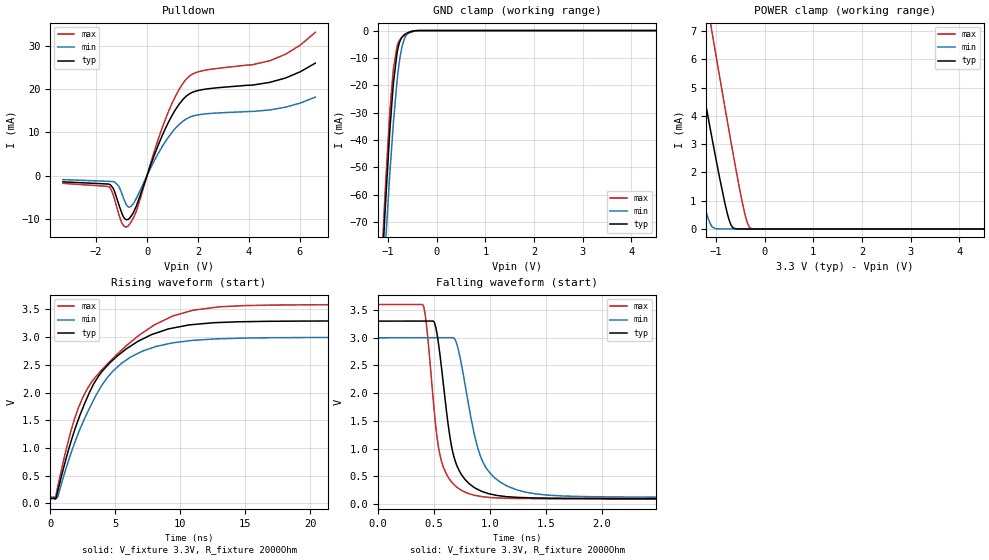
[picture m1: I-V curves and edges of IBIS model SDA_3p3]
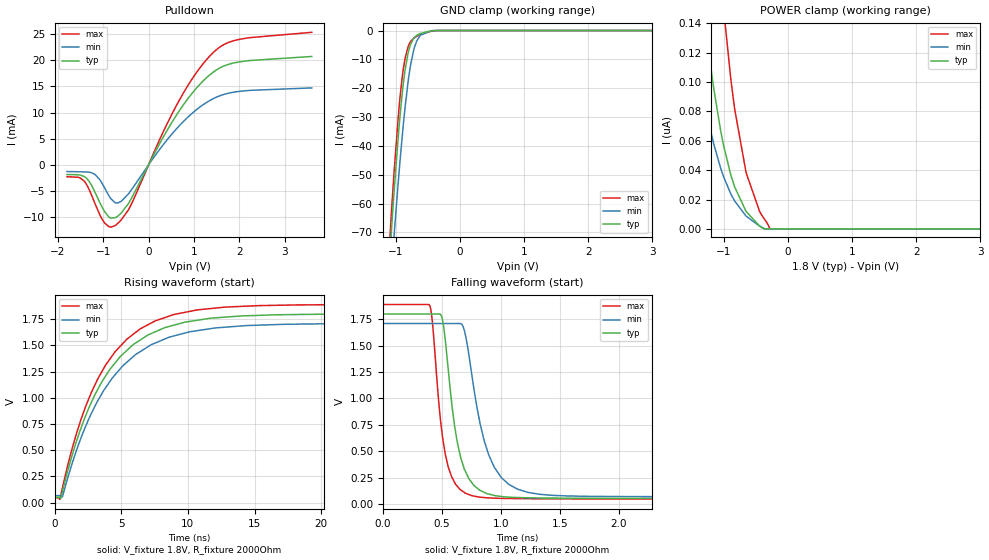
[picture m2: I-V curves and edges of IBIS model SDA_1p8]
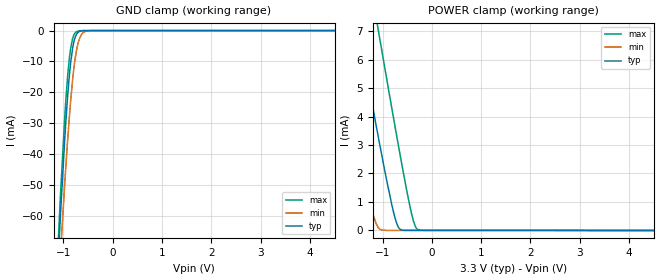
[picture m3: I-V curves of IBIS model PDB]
|Texas Instruments Incorporated
| Marketing part#   Digital Voltage Range   Package-type   #pins
| DS90UB940N-Q1   1.71V-3.6V   QFN   64
[IBIS Ver]   4.1
[File name]   ds90ub940n_q1.ibs
[File Rev]   1.0
[Date]   03/19/2019
[Source]
| Texas Instruments Incorporated.
| 12500 TI Blvd
| Dallas, TX -75243
[Notes]   Revision History:
| Rev 1.0: 03/19/2019
| - Initial version of the model
| - Model generated from simulations in TISPICE
| - C_comp although listed in numerical order of value are
|   obtained from varying PVT conditions. For PVT conditions for
|   each specific value refer the buffer description under
|   respective [Model]. IBIS model user is responsible for using
|   appropriate C_comp to simulate for Signal Integrity.
| - Warnings regarding combined Non-monotonicity of various models have been
|   reviewd and considered minor and can be ignored.
| - Model names with a trailing _1p8 contains the model for
|   1.8V operation.Model names with a trailing _3p3 contains the model
|   for 3.3V operation.
| - CSI driver depending on the mode of operation has two models,
|   csi_hs for high speed mode and csi_lp for low power mode.
[Disclaimer]
| This model is designed as an aid for customers of Texas Instruments.
| TI and its licensors and suppliers make no warranties, either expressed
| or implied, with respect to this  model, including the warranties of
| merchantability or fitness for a particular purpose. The model is
| provided solely on an "as is" basis. The entire risk as to its quality
| and performance is with the customer.
[Copyright]
 (C) Copyright 2014 Texas Instruments Incorporated.All rights reserved.
|   Device
[Component]   ds90ub940n_q1
[Manufacturer]   TI
[Package]  |QFN   64
|   typ   min   max
R_pkg   0.067   0.027   0.083
L_pkg   0.937nH   0.593nH   1.143nH
C_pkg   0.144pF   0.126pF   0.200pF
[Pin]  signal_name   model_name   R_pin   L_pin   C_pin
1   LOCK   GPIO   NA   NA   NA
2   CAP_12S   NC   NA   NA   NA
3   VDDIO   POWER   NA   NA   NA
4   BISTC/INTB   GPIO   NA   NA   NA
5   BISTEN   GPIO   NA   NA   NA
6   VDDL12_0   POWER   NA   NA   NA
7   SDOUT/GPIO0/PASS   GPIO   NA   NA   NA
8   SWC/GPIO1   GPIO   NA   NA   NA
9   I2S_DD/GPIO3   GPIO   NA   NA   NA
10   I2S_DC/GPIO2   GPIO   NA   NA   NA
11   I2S_DB/GPIO5   GPIO   NA   NA   NA
12   I2S_DA/GPIO6   GPIO   NA   NA   NA
13   I2S_CLK/GPIO8   GPIO   NA   NA   NA
14   I2S_WC/GPIO7   GPIO   NA   NA   NA
15   MCLK   GPIO   NA   NA   NA
16   D_GPIO3/SS   GPIO   NA   NA   NA
17   D_GPIO2/SPCK   GPIO   NA   NA   NA
18   D_GPIO1/MISO   GPIO   NA   NA   NA
19   D_GPIO0/MOSI   GPIO   NA   NA   NA
20   VDD12_LVD0   POWER   NA   NA   NA
21   CSI0_CLK-   CSI   NA   NA   NA
22   CSI0_CLK+   CSI   NA   NA   NA
23   CSI0_D0-   CSI   NA   NA   NA
24   CSI0_D0+   CSI   NA   NA   NA
25   CSI0_D1-   CSI   NA   NA   NA
26   CSI0_D1+   CSI   NA   NA   NA
27   CSI0_D2-   CSI   NA   NA   NA
28   CSI0_D2+   CSI   NA   NA   NA
29   CSI0_D3-   CSI   NA   NA   NA
30   CSI0_D3+   CSI   NA   NA   NA
31   VDD33_B   POWER   NA   NA   NA
32   VDD12_CSI   POWER   NA   NA   NA
33   VDD12_CSI1   POWER   NA   NA   NA
34   CSI1_CLK-   CSI   NA   NA   NA
35   CSI1_CLK+   CSI   NA   NA   NA
36   CSI1_D0-   CSI   NA   NA   NA
37   CSI1_D0+   CSI   NA   NA   NA
38   CSI1_D1-   CSI   NA   NA   NA
39   CSI1_D1+   CSI   NA   NA   NA
40   CSI1_D2-   CSI   NA   NA   NA
41   CSI1_D2+   CSI   NA   NA   NA
42   CSI1_D3-   CSI   NA   NA   NA
43   CSI1_D3+   CSI   NA   NA   NA
44   VDDL12_1   POWER   NA   NA   NA
45   I2C_SCL   SDA   NA   NA   NA
46   I2C_SDA   SDA   NA   NA   NA
47   IDX   NC   NA   NA   NA
48   PDB   PDB   NA   NA   NA
49   CAP_PLL0   NC   NA   NA   NA
50   MODE_SEL1   GPIO   NA   NA   NA
51   VDDP12_CH0   POWER   NA   NA   NA
52   VDDR12_CH0   POWER   NA   NA   NA
53   RIN0+   RX_CML_RCV   NA   NA   NA
54   RIN0-   RX_CML_RCV   NA   NA   NA
55   CMF   NC   NA   NA   NA
56   VDD33_A   POWER   NA   NA   NA
57   VDDR12_CH1   POWER   NA   NA   NA
58   RIN1+   RX_CML_RCV   NA   NA   NA
59   RIN-   RX_CML_RCV   NA   NA   NA
60   VDDP12_CH1   POWER   NA   NA   NA
61   MODE_SEL0   GPIO   NA   NA   NA
62   CMLOUTP   RX_CML   NA   NA   NA
63   CMLOUTN   RX_CML   NA   NA   NA
64   CAP_PLL1   NC   NA   NA   NA
[Diff pin]  inv_pin  vdiff  tdelay_typ  tdelay_min  tdelay_max
37   36   NA   NA   NA   NA
24   23   NA   NA   NA   NA
43   42   NA   NA   NA   NA
41   40   NA   NA   NA   NA
39   38   NA   NA   NA   NA
35   34   NA   NA   NA   NA
30   29   NA   NA   NA   NA
28   27   NA   NA   NA   NA
26   25   NA   NA   NA   NA
22   21   NA   NA   NA   NA
53   54   0.1   NA   NA   NA
58   59   0.1   NA   NA   NA
62   63   NA   NA   NA   NA
|   Model Selectors
[Model Selector]  GPIO
GPIO_3p3   I/O buffer in 3.3V mode
GPIO_1p8   I/O buffer in 1.8V mode
[Model Selector]  SDA
SDA_3p3   buffer in 3.3V mode
SDA_1p8   buffer in 1.8V mode
[Model Selector]  CSI
csi_hs   CSI high speed mode
csi_lp   CSI low power mode
| Models and submodels in the file (9): SDA_3p3 (I/O_open_drain), SDA_1p8 (I/O_open_drain), PDB (Input), GPIO_3p3 (I/O), GPIO_1p8 (I/O), RX_CML (Output), RX_CML_RCV (Input), csi_lp (Output), csi_hs (Output)
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|   Model
[Model]   SDA_3p3
Model_type   I/O_open_drain
Polarity   Non-Inverting
Enable   Active-Low
Vinl = 0.8
Vinh = 2.0
Vmeas = 1.65
Vref = 3.3
Cref = 1pF
Rref = 2000
|   typ   min   max
C_comp   0.9710pF   0.8915pF   1.0265pF
[Voltage Range]   3.3   3   3.6
[Temperature Range]   27   105   -40
[Pullup Reference]   3.3   3   3.6
[Pulldown Reference]   0   0   0
[Power Clamp Reference]   3.3   3   3.6
[GND Clamp Reference]   0   0   0
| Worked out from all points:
|   slope of the pulldown table from 0 to 0.495 V, typ, clamps not added: 63.1 ohm
|   GND clamp passes 1 mA (typ) near -0.62 V on its own axis
|   POWER clamp passes 1 mA (typ) near -0.83 V on its own axis
|   falling waveform, V_fixture 3.3V, R_fixture 2000Ohm: 20-80 % time 142ps typ, 200ps min, 116ps max; typ from 3.3 V to 0.094 V
|   rising waveform, V_fixture 3.3V, R_fixture 2000Ohm: 20-80 % time 3.99ns typ, 3.69ns min, 5.04ns max; typ from 0.094 V to 3.29 V
[Pulldown]
|   Voltage   I(typ)   I(min)   I(max)
-3.3V     -1.45mA    -925.3uA   -1.808mA
-1.508V   -1.967mA   -1.347mA   -2.522mA
-1.31V    -3.194mA   -1.421mA   -4.787mA
-1.102V   -6.774mA   -2.536mA   -9.092mA
-815.1mV  -10.25mA   -6.717mA   -11.95mA
-676.5mV  -9.81mA    -7.294mA   -11.2mA
-429mV    -7.201mA   -5.395mA   -8.4mA
788.7mV   11.74mA    8.476mA    14.06mA
1.541V    18.41mA    13.12mA    22.35mA
2.115V    19.85mA    14.17mA    24.2mA
4.818V    21.59mA    15.2mA     26.6mA
6.6V      26.05mA    18.16mA    33.18mA
[GND Clamp]
|   Voltage   I(typ)   I(min)   I(max)
-3.3V     -902.9mA   -825.4mA   -957.5mA
-1.152V   -98.03mA   -109.4mA   -93.38mA
-1.073V   -70.75mA   -84.7mA    -64.47mA
-1.053V   -64.23mA   -78.71mA   -57.66mA
-963.6mV  -37.33mA   -53.07mA   -30.46mA
-884.4mV  -18.7mA    -33.03mA   -13.6mA
-815.1mV  -8.486mA   -18.9mA    -6.02mA
-745.8mV  -3.591mA   -9.168mA   -3.158mA
-676.5mV  -1.732mA   -3.801mA   -2.041mA
-597.3mV  -846.9uA   -1.184mA   -1.233mA
-290.4mV  -1.142uA   -1.534uA   -2.038uA
6.6V      0A         0A         0A
[POWER Clamp]
|   Voltage   I(typ)   I(min)   I(max)
-3.3V     24.9mA     18.55mA    29.99mA
-1.973V   11.79mA    6.871mA    16.19mA
-1.538V   7.556mA    3.177mA    11.67mA
-1.419V   6.415mA    2.213mA    10.44mA
-1.181V   4.162mA    499.6uA    8.007mA
-1.092V   3.334mA    113.7uA    7.1mA
-1.013V   2.611mA    13.4uA     6.297mA
-815.1mV  915.8uA    553.8nA    4.314mA
-686.4mV  134uA      391.9nA    3.052mA
-419.1mV  567.3nA    222.4nA    641.7uA
-280.5mV  431.6nA    163.3nA    23.14uA
6.6V      0A         0A         0A
[Ramp]
R_load = 2000
|   typ   min   max
dV/dt_r   1.91865/3.99467e-09   1.72713/3.68665e-09   2.10002/5.03843e-09
dV/dt_f   1.92346/1.41684e-10   1.73016/2.00104e-10   2.10724/1.15619e-10
[Falling Waveform]
V_fixture = 3.3V
V_fixture_min = 3V
V_fixture_max = 3.6V
R_fixture = 2000Ohm
C_fixture = 0F
|   Time   V(typ)   V(min)   V(max)
0s        3.299V     3V         3.598V
401.2ps   3.3V       3V         3.589V
495.7ps   3.296V     3.001V     1.794V
535.3ps   2.947V     3.001V     1.069V
623.9ps   1.453V     3.001V     491.6mV
685.1ps   798.2mV    2.975V     338.8mV
886.9ps   268.7mV    1.035V     149.6mV
1.014ns   176.8mV    528.8mV    116.6mV
2.022ns   101.4mV    131.1mV    91.92mV
30ns      93.69mV    116.1mV    86.39mV
[Rising Waveform]
V_fixture = 3.3V
V_fixture_min = 3V
V_fixture_max = 3.6V
R_fixture = 2000Ohm
C_fixture = 0F
|   Time   V(typ)   V(min)   V(max)
0s        93.65mV    116mV      86.22mV
359.9ps   91.18mV    116.4mV    75.06mV
561.3ps   205.6mV    113.6mV    286.4mV
1.611ns   1.129V     918.4mV    1.323V
2.779ns   1.875V     1.6V       2.04V
3.7ns     2.292V     2.024V     2.339V
4.786ns   2.579V     2.377V     2.607V
8.024ns   3.062V     2.822V     3.221V
13.04ns   3.262V     2.968V     3.545V
30ns      3.291V     2.995V     3.586V
|   Model
[Model]   SDA_1p8
Model_type   I/O_open_drain
Polarity   Non-Inverting
Enable   Active-Low
Vinl = 0.63
Vinh = 1.17
Vmeas = 0.9
Vref = 1.8
Cref = 1pF
Rref = 2000
|   typ   min   max
C_comp   0.9710pF   0.8915pF   1.0265pF
[Voltage Range]   1.8   1.71   1.89
[Temperature Range]   27   105   -40
[Pullup Reference]   1.8   1.71   1.89
[Pulldown Reference]   0   0   0
[Power Clamp Reference]   1.8   1.71   1.89
[GND Clamp Reference]   0   0   0
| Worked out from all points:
|   slope of the pulldown table from 0 to 0.27 V, typ, clamps not added: 60.4 ohm
|   GND clamp passes 1 mA (typ) near -0.61 V on its own axis
|   falling waveform, V_fixture 1.8V, R_fixture 2000Ohm: 20-80 % time 132ps typ, 193ps min, 106ps max; typ from 1.8 V to 0.051 V
|   rising waveform, V_fixture 1.8V, R_fixture 2000Ohm: 20-80 % time 4.21ns typ, 4.43ns min, 4.04ns max; typ from 0.051 V to 1.8 V
[Pulldown]
|   Voltage   I(typ)   I(min)   I(max)
-1.8V     -1.859mA   -1.287mA   -2.282mA
-1.417V   -2.271mA   -1.364mA   -3.165mA
-1.19V    -5.134mA   -1.813mA   -7.284mA
-973.8mV  -8.941mA   -4.387mA   -11.13mA
-736.2mV  -10.14mA   -7.276mA   -11.64mA
-444.6mV  -7.432mA   -5.576mA   -8.646mA
311.4mV   5.124mA    3.727mA    6.101mA
689.4mV   10.5mA     7.592mA    12.55mA
1.37V     17.37mA    12.41mA    21.01mA
1.672V    18.97mA    13.51mA    23.08mA
1.975V    19.66mA    14.03mA    23.97mA
3.6V      20.75mA    14.73mA    25.38mA
[GND Clamp]
|   Voltage   I(typ)   I(min)   I(max)
-1.8V     -344.1mA   -328mA     -357.8mA
-1.195V   -113.6mA   -123.4mA   -110.1mA
-1.066V   -68.46mA   -82.6mA    -62.07mA
-1.028V   -56.28mA   -71.3mA    -49.43mA
-936mV    -30.12mA   -45.72mA   -23.62mA
-892.8mV  -20.35mA   -34.99mA   -14.97mA
-855mV    -13.62mA   -26.56mA   -9.617mA
-768.6mV  -4.745mA   -11.85mA   -3.791mA
-671.4mV  -1.655mA   -3.543mA   -1.983mA
-617.4mV  -1.022mA   -1.614mA   -1.421mA
-412.2mV  -38.78uA   -33.09uA   -88.67uA
3.6V      0A         0A         0A
[POWER Clamp]
|   Voltage   I(typ)   I(min)   I(max)
-1.8V     458.9nA    280.6nA    904.5nA
-1.503V   243.7nA    144.2nA    525.8nA
-1.341V   162.3nA    96.31nA    372.4nA
-1.238V   121.5nA    72.76nA    290.9nA
-1.157V   94.86nA    57.44nA    234.9nA
-1.006V   56.75nA    35.51nA    149.9nA
-838.8mV  29.27nA    19.4nA     83.29nA
-655.2mV  11.89nA    8.694nA    38.26nA
-444.6mV  1.962nA    1.974nA    11.96nA
-379.8mV  101pA      411.1pA    7.355nA
-277.2mV  0A         0A         0A
3.6V      0A         0A         0A
[Ramp]
R_load = 2000
|   typ   min   max
dV/dt_r   1.0493/4.21176e-09   0.986343/4.42759e-09   1.10673/4.03919e-09
dV/dt_f   1.04951/1.32131e-10   0.986624/1.92728e-10   1.10694/1.05856e-10
[Falling Waveform]
V_fixture = 1.8V
V_fixture_min = 1.71V
V_fixture_max = 1.89V
R_fixture = 2000Ohm
C_fixture = 0F
|   Time   V(typ)   V(min)   V(max)
0s        1.8V       1.71V      1.89V
399ps     1.8V       1.71V      1.875V
495.9ps   1.782V     1.71V      715.4mV
551.4ps   1.295V     1.71V      358.3mV
656.5ps   449.1mV    1.709V     135.4mV
705ps     295mV      1.569V     100.1mV
883.1ps   98.69mV    512mV      59.03mV
1.141ns   62.07mV    140.9mV    51.9mV
1.728ns   55.42mV    73.69mV    48.83mV
30ns      50.75mV    65.56mV    45.02mV
[Rising Waveform]
V_fixture = 1.8V
V_fixture_min = 1.71V
V_fixture_max = 1.89V
R_fixture = 2000Ohm
C_fixture = 0F
|   Time   V(typ)   V(min)   V(max)
0s        50.76mV    65.51mV    45.01mV
375.8ps   46.57mV    66.04mV    30.65mV
577.9ps   105.3mV    57.79mV    142.6mV
1.967ns   709.3mV    616mV      792mV
3.806ns   1.205V     1.094V     1.309V
5.402ns   1.45V      1.337V     1.558V
7.556ns   1.63V      1.523V     1.734V
10.11ns   1.728V     1.629V     1.823V
14.38ns   1.782V     1.688V     1.874V
30ns      1.8V       1.709V     1.89V
|   Model
[Model]   PDB
Model_type   Input
Vinl = 0.8
Vinh = 2.0
|   typ   min   max
C_comp   0.8892pF   0.8437pF   0.9472pF
[Voltage Range]   3.3   3   3.6
[Temperature Range]   27   105   -40
[Power Clamp Reference]   3.3   3   3.6
[GND Clamp Reference]   0   0   0
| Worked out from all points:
|   GND clamp passes 1 mA (typ) near -0.72 V on its own axis
|   POWER clamp passes 1 mA (typ) near -0.82 V on its own axis
[GND Clamp]
|   Voltage   I(typ)   I(min)   I(max)
-3.3V     -832.2mA   -757.4mA   -879.9mA
-1.152V   -89.06mA   -98.92mA   -84.43mA
-1.073V   -63.87mA   -76.27mA   -57.71mA
-1.053V   -57.85mA   -70.79mA   -51.39mA
-963.6mV  -32.95mA   -47.39mA   -25.88mA
-914.1mV  -21.37mA   -35.62mA   -14.86mA
-884.4mV  -15.54mA   -29.14mA   -9.781mA
-805.2mV  -5.059mA   -14.8mA    -2.192mA
-716.1mV  -829.7uA   -5.061mA   -225.6uA
-617.1mV  -67.97uA   -964.1uA   -15.09uA
-448.8mV  -2.962uA   -23.21uA   -2.979uA
6.6V      0A         0A         0A
[POWER Clamp]
|   Voltage   I(typ)   I(min)   I(max)
-3.3V     24.7mA     18.42mA    29.8mA
-2.231V   14.24mA    9.067mA    18.74mA
-1.944V   11.46mA    6.592mA    15.79mA
-1.488V   7.066mA    2.767mA    11.11mA
-1.231V   4.624mA    808.9uA    8.492mA
-1.092V   3.334mA    114.8uA    7.088mA
-1.053V   2.971mA    42.82uA    6.689mA
-815.1mV  918.5uA    2.23uA     4.315mA
-686.4mV  137.1uA    2.126uA    3.055mA
-419.1mV  3.78uA     1.983uA    646.4uA
-280.5mV  3.652uA    1.926uA    28.14uA
6.6V      0A         0A         0A
